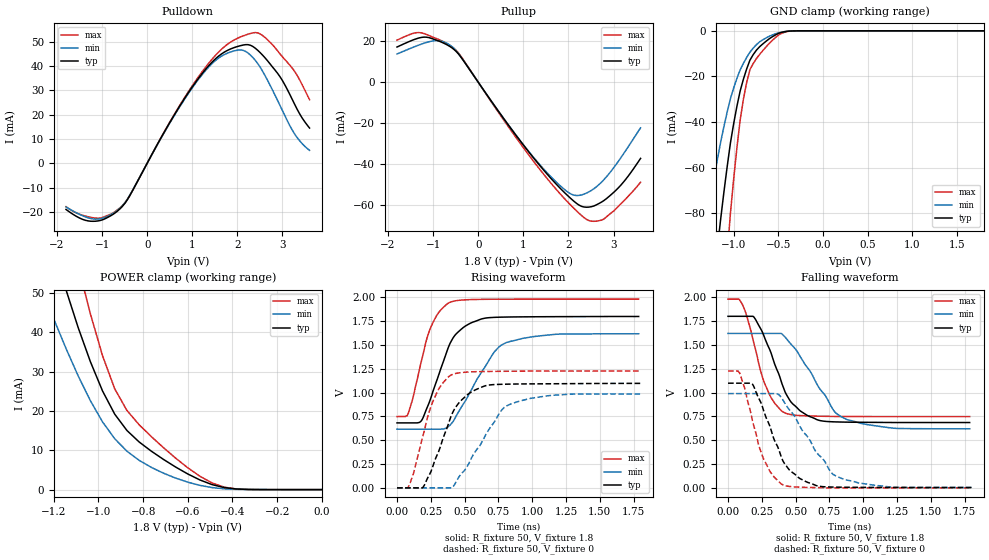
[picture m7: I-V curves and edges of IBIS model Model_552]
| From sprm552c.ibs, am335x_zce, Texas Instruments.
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| Model based on original model for BCSHTLTCSCDDVPBFZ_SSDHV
|   Sub model SR10_12MA_PADP_10PER_1P8
[model]   Model_552
|[Description]  [1.8V-3-STATE-NOTERM-SR10:12MA, IND, 10%]
|   Fast slew rate (SR[1:0] = "10"), 0.67 * RExt = 1.500 * Iout
|   (I[2:0] = "111"), 12mA nominal with Rext = 50R,ODT off (ODT[1:0]
|   = "00") CMOS mode,Industrial temperature range (-40C to 125C,
|   25C nominal),10% power supply tolerance
|[Input Load]   NOTERM
|[Output Drive] SR10:12MA
|Voltage   1.8V
|Mode   3-STATE
Model_type   3-state
Polarity   Non-Inverting
Enable   Active-Low
Cref =  15pF
Rref =  100.0000M
Vref =  0V
Vmeas =  0.9
C_comp   1.851324p   1.663768p   1.973575p
[Temperature Range]   25   125   -40
[Voltage Range]   1.8   1.62   1.98
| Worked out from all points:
|   slope of the pulldown table from 0 to 0.27 V, typ, clamps not added: 29.2 ohm
|   slope of the pullup table from 0 to 0.27 V, typ, clamps not added: 31.3 ohm
|   GND clamp passes 1 mA (typ) near -0.49 V on its own axis
|   POWER clamp passes 1 mA (typ) near -0.47 V on its own axis
|   rising waveform, R_fixture 50, V_fixture 1.8: 20-80 % time 175ps typ, 252ps min, 139ps max; typ from 0.682 V to 1.8 V
|   rising waveform, R_fixture 50, V_fixture 0: 20-80 % time 186ps typ, 254ps min, 151ps max; typ from 0 V to 1.1 V
|   falling waveform, R_fixture 50, V_fixture 1.8: 20-80 % time 192ps typ, 261ps min, 150ps max; typ from 1.8 V to 0.685 V
|   falling waveform, R_fixture 50, V_fixture 0: 20-80 % time 188ps typ, 274ps min, 150ps max; typ from 1.1 V to 0.004 V
[POWER_clamp]
-1.8V     194.9mA    137.1mA    262.8mA
-1.236V   68.49mA    48.51mA    92.67mA
-1.145V   50.76mA    35.86mA    69.65mA
-1.127V   47.56mA    33.54mA    65.34mA
-1.055V   35.4mA     24.69mA    48.69mA
-981.8mV  25.06mA    17.2mA     34.01mA
-927.3mV  19.17mA    12.93mA    25.61mA
-872.7mV  15.03mA    9.767mA    20.12mA
-818.2mV  12.12mA    7.45mA     16.5mA
-654.5mV  5.738mA    2.93mA     8.003mA
-436.4mV  508.2uA    199.4uA    613uA
0V        2.273nA    15.95nA    16.67nA
[Pulldown]
-1.8V     -19.04mA   -18.02mA   -17.88mA
-1.145V   -23.87mA   -23.03mA   -22.59mA
-545.5mV  -17.69mA   -17.39mA   -17.39mA
545.5mV   18.16mA    17.9mA     18.33mA
1.091V    33.8mA     33.39mA    34.37mA
1.527V    43.21mA    42.5mA     44.68mA
1.964V    47.83mA    46.41mA    51.1mA
2.291V    48.55mA    44.5mA     53.43mA
2.618V    43.28mA    35.9mA     51.68mA
2.945V    35.6mA     23.75mA    44.98mA
3.218V    26.2mA     13.58mA    39.11mA
3.6V      14.49mA    5.303mA    26.15mA
[Pullup]
-1.8V     17.15mA    13.74mA    20.51mA
-1.309V   21.6mA     18.18mA    24.22mA
-927.3mV  20.52mA    20.27mA    21.29mA
-600mV    17.03mA    17.65mA    17.57mA
-381.8mV  12.19mA    12.29mA    12.62mA
1.2V      -36.27mA   -35.99mA   -37.86mA
1.745V    -50.17mA   -49.12mA   -52.76mA
2.127V    -58.27mA   -55.22mA   -61.77mA
2.455V    -61.03mA   -53.58mA   -67.59mA
2.727V    -58.68mA   -48.99mA   -67.43mA
3.164V    -50.29mA   -36.88mA   -59.41mA
3.6V      -37.24mA   -22.35mA   -48.89mA
[GND_clamp]
-1.8V     -346.1mA   -209.3mA   -568.3mA
-1.327V   -149.7mA   -89.03mA   -250.9mA
-1.291V   -135.6mA   -80.47mA   -227.5mA
-1.145V   -82.35mA   -48.67mA   -137.7mA
-1.073V   -59.44mA   -35.55mA   -97.96mA
-1.036V   -49.1mA    -29.72mA   -79.9mA
-927.3mV  -26.31mA   -17.11mA   -38.99mA
-854.5mV  -16.67mA   -11.64mA   -22.56mA
-818.2mV  -12.86mA   -9.351mA   -16.98mA
-672.7mV  -5.705mA   -3.913mA   -8.624mA
-381.8mV  -120.4uA   -129uA     -167.4uA
1.8V      2.273nA    454nA      6.646nA
[Ramp]
dV/dt_f 0.67354381/0.19374836n 0.60493045/0.26294605n 0.74101501/0.15024182n
dV/dt_r 0.66131926/0.18702299n 0.59647099/0.25504485n 0.73710779/0.1509299n
R_load = 50
[Rising Waveform]
R_fixture = 50
V_fixture = 1.8
V_fixture_min = 1.62
V_fixture_max = 1.98
0s        681.6mV    615.9mV    748.1mV
84.8ps    681.6mV    615.9mV    786.5mV
182.4ps   708.8mV    615.9mV    1.342V
266.6ps   1.016V     615.9mV    1.736V
387.8ps   1.502V     652.5mV    1.944V
547.5ps   1.731V     1.022V     1.975V
721.2ps   1.789V     1.429V     1.979V
809.8ps   1.792V     1.526V     1.98V
1.179ns   1.796V     1.612V     1.98V
1.787ns   1.798V     1.617V     1.98V
[Rising Waveform]
R_fixture = 50
V_fixture = 0
V_fixture_min = 0
V_fixture_max = 0
0s        0V         0V         0V
80.5ps    0V         0V         0V
123.4ps   0V         0V         159.2mV
191.8ps   5.122mV    0V         544.2mV
295.5ps   341.8mV    0V         1.002V
405.6ps   772.2mV    0V         1.188V
557.6ps   1.012V     332.8mV    1.217V
821.9ps   1.088V     868.3mV    1.224V
1.144ns   1.092V     970.5mV    1.225V
1.801ns   1.096V     985mV      1.226V
[Falling Waveform]
R_fixture = 50
V_fixture = 1.8
V_fixture_min = 1.62
V_fixture_max = 1.98
0s        1.799V     1.619V     1.979V
103.7ps   1.799V     1.619V     1.931V
192ps     1.79V      1.619V     1.512V
254.9ps   1.631V     1.619V     1.161V
309.7ps   1.446V     1.619V     969.5mV
422.1ps   1.005V     1.582V     784.4mV
591.4ps   755.7mV    1.253V     754.6mV
837.4ps   690.2mV    745.5mV    748.5mV
1.237ns   685.1mV    624mV      747.3mV
1.787ns   684.9mV    619.3mV    747.2mV
[Falling Waveform]
R_fixture = 50
V_fixture = 0
V_fixture_min = 0
V_fixture_max = 0
0s        1.098V     988.7mV    1.225V
86.6ps    1.098V     988.7mV    1.203V
180.9ps   1.087V     988.7mV    702.3mV
262.4ps   814.2mV    988.7mV    305.3mV
321ps     594.7mV    988.7mV    151.3mV
403.1ps   291.8mV    928.3mV    33.78mV
575.4ps   66.05mV    557.3mV    4.99mV
808.2ps   7.44mV     116.9mV    0V
1.196ns   3.994mV    8.763mV    0V
1.801ns   3.836mV    4.099mV    0V
